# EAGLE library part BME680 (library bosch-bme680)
BME680 integrates for the first time individual high linearity and high accuracy sensors for gas, pressure, humidity and temperature. The library has been designed by Richard Magdycz
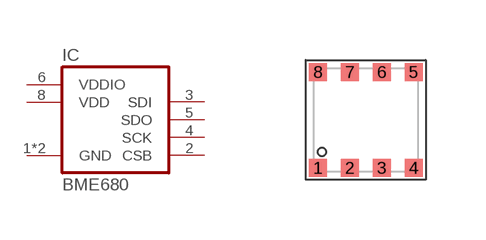
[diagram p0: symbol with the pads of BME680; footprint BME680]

Designator prefix IC

## BME680  [BME680]
1  GND  pwr
2  CSB  in
3  SDI  in
4  SCK  in
5  SDO  out
6  VDDIO  pwr
7  GND  pwr
8  VDD  pwr

## Footprint BME680 (pad centres in mm)
smd 0.45 x 0.45: 1 -1.2,-1.2; 2 -0.4,-1.2; 3 0.4,-1.2; 4 1.2,-1.2; 5 1.2,1.2; 6 0.4,1.2; 7 -0.4,1.2; 8 -1.2,1.2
